(* Logix 5000 Rung export; software revision 16.03 *)

TYPE MNETClockType :   // Allows read/write of clock value between the module and processor
STRUCT
   Read : BOOL;   // Reads current time from the module
   Write : BOOL;   // Writes current time from the module
   Config : MNETDateTime;   // Date and time configuration read or written between the module and processor
END_STRUCT
END_TYPE

TYPE MNETDateTime :   // Stores the date and time value
STRUCT
   Year : DINT;
   Month : DINT;
   Day : DINT;
   Hour : DINT;
   Minute : DINT;
   Seconds : DINT;
END_STRUCT
END_TYPE

TYPE MNETEthernet :   // Stores the MVI56E-MNETR IP settings
STRUCT
   IP : INT[4];
   Netmask : INT[4];
   Gateway : INT[4];
END_STRUCT
END_TYPE

TYPE MNETEthernetType :   // Allows read/write Ethernet settings between the module and processor
STRUCT
   Read : BOOL;   // Enable Ethernet configuration transfer from module to processor
   Write : BOOL;   // Enable Ethernet configuration transfer from processor to module
   Config : MNETEthernet;
END_STRUCT
END_TYPE

ADD_ON_INSTRUCTION AOI56MNET_Optional   (* revision 1.0 *)
// MVI56-MNET Optional Add-On Ethernet/Clock
// Revision note:
// Release
VAR_IN_OUT
   MVI56MNETEthernet : MNETEthernetType; {required}   // MVI56E-MNET Rev2 Ethernet Settings
   MVI56MNETClock : MNETClockType; {required}   // MVI56E-MNET Rev2 Clock Settings
   ReadEthernetMSG : MESSAGE; {required}   // Read Ethernet Settings Message
   WriteEthernetMSG : MESSAGE; {required}   // Write Ethernet Settings Message
   ReadClockMSG : MESSAGE; {required}   // Read Clock Settings Message
   WriteClockMSG : MESSAGE; {required}   // Write Clock Settings Message
END_VAR

ROUTINE Logic   (* ladder *)
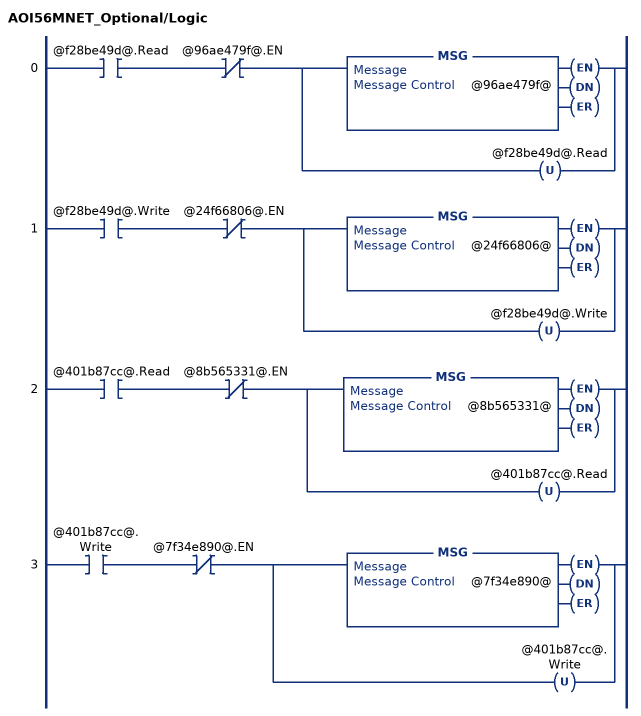
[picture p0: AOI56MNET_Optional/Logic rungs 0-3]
   0: XIC(@f28be49d@.Read)XIO(@96ae479f@.EN)[MSG(@96ae479f@) ,OTU(@f28be49d@.Read) ];
   1: XIC(@f28be49d@.Write)XIO(@24f66806@.EN)[MSG(@24f66806@) ,OTU(@f28be49d@.Write) ];
   2: XIC(@401b87cc@.Read)XIO(@8b565331@.EN)[MSG(@8b565331@) ,OTU(@401b87cc@.Read) ];
   3: XIC(@401b87cc@.Write)XIO(@7f34e890@.EN)[MSG(@7f34e890@) ,OTU(@401b87cc@.Write) ];
END_ROUTINE
END_ADD_ON_INSTRUCTION

VAR_GLOBAL   (* controller tags *)
   WriteClockMSG : MESSAGE;
        MessageParameters(MessageType := CIP Generic, RequestedLength := 24, ConnectedFlag := 2, ConnectionPath := MNET, ServiceCode := 16#0010, ObjectType := 16#0004, TargetObject := 8, AttributeNumber := 16#0020, LocalElement := MVI56EMNETClock.Config)
   MVI56EMNETClock : MNETClockType;
   MVI56EMNETEthernet : MNETEthernetType;
   ReadEthernetMSG : MESSAGE;
        MessageParameters(MessageType := CIP Generic, ConnectedFlag := 2, ConnectionPath := MNET, ServiceCode := 16#000e, ObjectType := 16#0004, TargetObject := 8, DestinationTag := MVI56EMNETEthernet.Config)
   ReadClockMSG : MESSAGE;
        MessageParameters(MessageType := CIP Generic, ConnectedFlag := 2, ConnectionPath := MNET, ServiceCode := 16#000e, ObjectType := 16#0004, TargetObject := 8, AttributeNumber := 16#0020, DestinationTag := MVI56EMNETClock.Config)
   AOI56EMNET_Optional : AOI56MNET_Optional;
   WriteEthernetMSG : MESSAGE;
        MessageParameters(MessageType := CIP Generic, RequestedLength := 24, ConnectedFlag := 2, ConnectionPath := MNET, ServiceCode := 16#0010, ObjectType := 16#0004, TargetObject := 8, LocalElement := MVI56EMNETEthernet.Config)
END_VAR

PROGRAM MainProgram

ROUTINE MainRoutine   (* ladder *)
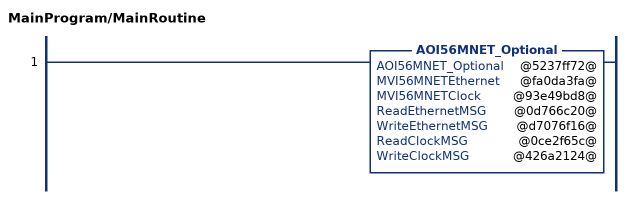
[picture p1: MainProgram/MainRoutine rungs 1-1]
   1: AOI56MNET_Optional(@5237ff72@,@fa0da3fa@,@93e49bd8@,@0d766c20@,@d7076f16@,@0ce2f65c@,@426a2124@);
END_ROUTINE
END_PROGRAM
